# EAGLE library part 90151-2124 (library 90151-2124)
Headers & Wire Housings C-Grid PCB Conn DR Vt Tn-A 24Ckt Source: Datasheet
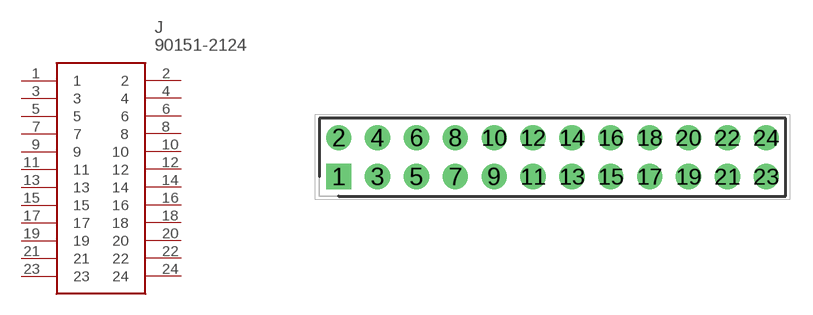
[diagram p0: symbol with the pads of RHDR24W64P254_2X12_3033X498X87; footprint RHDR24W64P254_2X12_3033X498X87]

Designator prefix J

## 90151-2124 (Description: Headers & Wire Housings C-Grid PCB Conn DR Vt Tn-A 24Ckt; Height: 8.7mm; Manufacturer_Name: Molex; Manufacturer_Part_Number: 90151-2124)  [RHDR24W64P254_2X12_3033X498X87]
1  1
2  2
3  3
4  4
5  5
6  6
7  7
8  8
9  9
10  10
11  11
12  12
13  13
14  14
15  15
16  16
17  17
18  18
19  19
20  20
21  21
22  22
23  23
24  24

## Footprint RHDR24W64P254_2X12_3033X498X87 (pad centres in mm)
90151-2124
drill 1.1 pad 1.65 square: 1 0,0
drill 1.1 pad 1.65: 2 0,2.54; 3 2.54,0; 4 2.54,2.54; 5 5.08,0; 6 5.08,2.54; 7 7.62,0; 8 7.62,2.54; 9 10.16,0; 10 10.16,2.54; 11 12.7,0; 12 12.7,2.54; 13 15.24,0; 14 15.24,2.54; 15 17.78,0; 16 17.78,2.54; 17 20.32,0; 18 20.32,2.54; 19 22.86,0; 20 22.86,2.54; 21 25.4,0; 22 25.4,2.54; 23 27.94,0; 24 27.94,2.54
